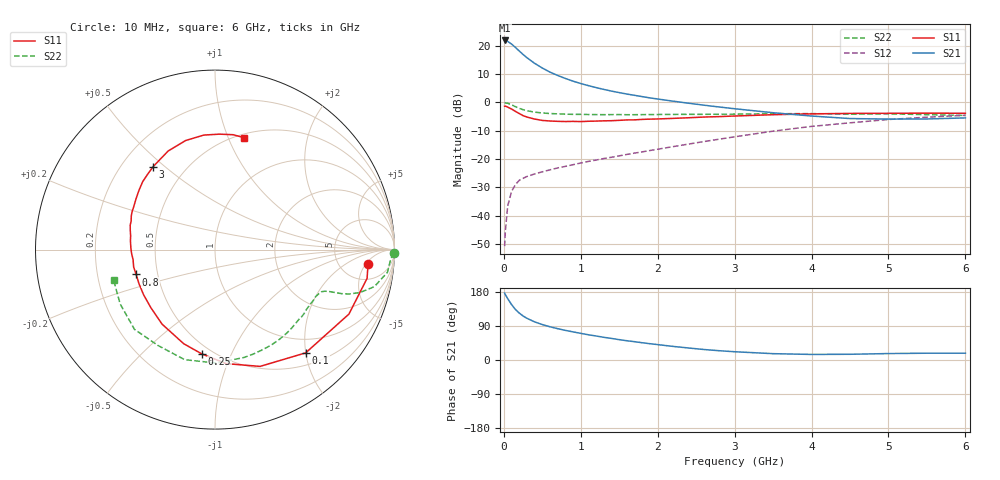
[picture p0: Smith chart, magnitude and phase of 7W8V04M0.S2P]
! Infineon Technologies  Discrete & RF Semiconductors
! BFS17W
! Si NPN RF Bipolar Junction Transistor in SOT323
! VCE = 8 V  IC = 4 mA
! Common Emitter S-Parameters:  August  1999
# GHz  S  MA  R  50
!  f  S11  S21  S12  S22
! GHz  MAG  ANG  MAG  ANG  MAG  ANG  MAG  ANG
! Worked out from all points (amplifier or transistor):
!   36 points, 10 MHz to 6 GHz, reference 50 ohm
!   highest |S21| = 21.9 dB at 10 MHz (marker M1)
!   |S21| within 3 dB of that: start of sweep to 171.8 MHz
!   unconditionally stable (mu >= 1): 653.8 MHz to 2.433 GHz; 5.116 GHz to end of sweep
!   at 250 MHz: K = 0.51, MSG = 21.9 dB, |S12| = -26.8 dB
!   at 1.4 GHz: K = 1.22, MAG = 8.8 dB, |S12| = -19.3 dB
!   at 6 GHz: K = 1.06, MAG = -1.9 dB, |S12| = -4.5 dB
!   S11 on the Smith chart (normalised r, x): 10 MHz: 10, -6; 100 MHz: 0.72, -2.00; 250 MHz: 0.44, -0.78; 800 MHz: 0.38, -0.13; 3 GHz: 0.33, +0.46; 6 GHz: 0.53, +1.14
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0.01  0.8566 -5.2  12.45 176.7  0.0029 81.2  0.9973 -1.1
0.02  0.8623 -10.7  12.4 172.5  0.0054 85.5  0.9808 -3.0
0.05  0.8282 -25.7  11.97 161.8  0.0148 78.1  0.9691 -7.5
0.1  0.7657 -48.7  10.77 146.4  0.0268 67.0  0.9114 -13.1
0.15  0.6975 -68.9  9.39 133.5  0.0353 59.1  0.8422 -16.5
0.2  0.6383 -84.4  8.125 123.9  0.0422 54.6  0.7881 -18.3
0.25  0.5858 -97.2  7.042 116.2  0.0457 50.6  0.7459 -19.2
0.3  0.5526 -108.4  6.178 110.1  0.0493 49.5  0.7157 -19.6
0.4  0.5093 -125.4  4.915 100.6  0.0547 49.0  0.675 -20.2
0.5  0.482 -137.9  4.057 93.5  0.0596 49.7  0.6528 -20.8
0.6  0.4707 -147.7  3.435 87.7  0.0647 51.0  0.6381 -21.6
0.8  0.4608 -162.5  2.655 78.2  0.0744 54.6  0.6222 -24.3
0.9  0.4635 -168.0  2.379 74.2  0.0797 56.4  0.6169 -25.7
1.1  0.4659 -178.0  1.982 66.5  0.0911 59.3  0.6126 -29.3
1.3  0.4739 173.9  1.702 59.9  0.1024 61.9  0.6089 -33.3
1.6  0.4919 163.8  1.408 50.8  0.121 64.9  0.6081 -39.6
2.2  0.5238 147.0  1.055 35.9  0.166 69.8  0.6154 -54.1
3  0.5767 126.7  0.775 21.8  0.2476 70.2  0.6224 -75.0
3.5  0.6082 115.4  0.659 16.7  0.3115 67.4  0.6322 -89.4
4.5  0.6411 95.6  0.52 15.1  0.4371 55.9  0.6214 -120.7
5.5  0.6479 81.1  0.511 17.9  0.5497 42.5  0.609 -150.2
6  0.6444 75.6  0.534 17.9  0.5937 35.8  0.5898 -163.4
